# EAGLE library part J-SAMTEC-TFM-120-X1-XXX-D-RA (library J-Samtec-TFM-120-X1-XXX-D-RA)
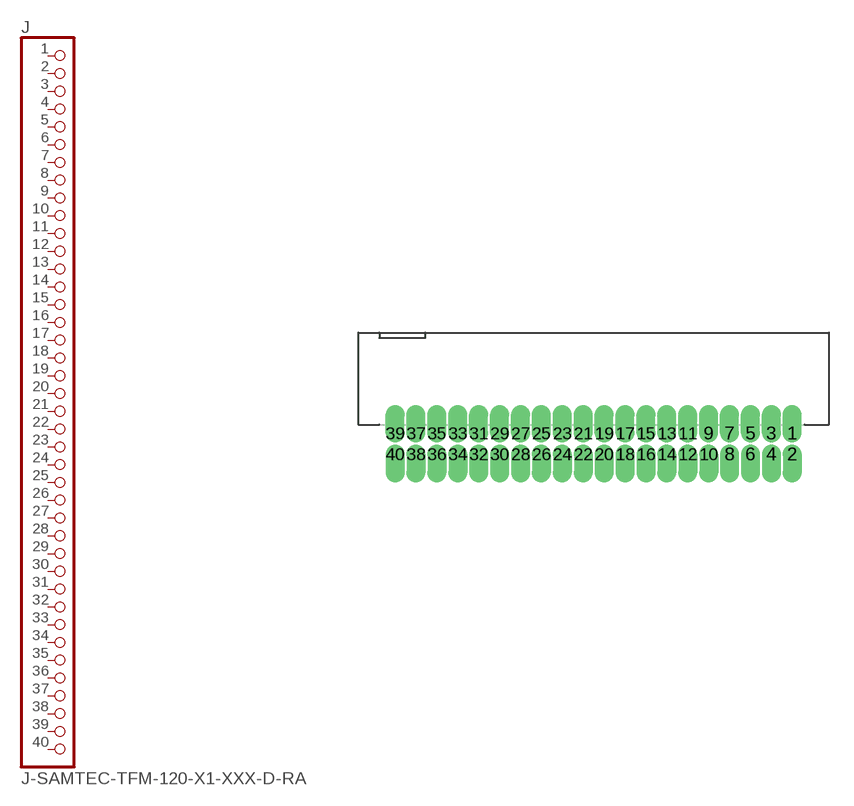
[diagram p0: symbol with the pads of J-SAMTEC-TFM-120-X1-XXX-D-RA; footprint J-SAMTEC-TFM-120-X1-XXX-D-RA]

Designator prefix J

## J-SAMTEC-TFM-120-X1-XXX-D-RA  [J-SAMTEC-TFM-120-X1-XXX-D-RA]
1  1  pas
2  2  pas
3  3  pas
4  4  pas
5  5  pas
6  6  pas
7  7  pas
8  8  pas
9  9  pas
10  10  pas
11  11  pas
12  12  pas
13  13  pas
14  14  pas
15  15  pas
16  16  pas
17  17  pas
18  18  pas
19  19  pas
20  20  pas
21  21  pas
22  22  pas
23  23  pas
24  24  pas
25  25  pas
26  26  pas
27  27  pas
28  28  pas
29  29  pas
30  30  pas
31  31  pas
32  32  pas
33  33  pas
34  34  pas
35  35  pas
36  36  pas
37  37  pas
38  38  pas
39  39  pas
40  40  pas

## Footprint J-SAMTEC-TFM-120-X1-XXX-D-RA (pad centres in mm)
drill 0.635 pad 0.965 offset: 1 12.065,0.635; 2 12.065,-0.635; 3 10.795,0.635; 4 10.795,-0.635; 5 9.525,0.635; 6 9.525,-0.635; 7 8.255,0.635; 8 8.255,-0.635; 9 6.985,0.635; 10 6.985,-0.635; 11 5.715,0.635; 12 5.715,-0.635; 13 4.445,0.635; 14 4.445,-0.635; 15 3.175,0.635; 16 3.175,-0.635; 17 1.905,0.635; 18 1.905,-0.635; 19 0.635,0.635; 20 0.635,-0.635; 21 -0.635,0.635; 22 -0.635,-0.635; 23 -1.905,0.635; 24 -1.905,-0.635; 25 -3.175,0.635; 26 -3.175,-0.635; 27 -4.445,0.635; 28 -4.445,-0.635; 29 -5.715,0.635; 30 -5.715,-0.635; 31 -6.985,0.635; 32 -6.985,-0.635; 33 -8.255,0.635; 34 -8.255,-0.635; 35 -9.525,0.635; 36 -9.525,-0.635; 37 -10.795,0.635; 38 -10.795,-0.635; 39 -12.065,0.635; 40 -12.065,-0.635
